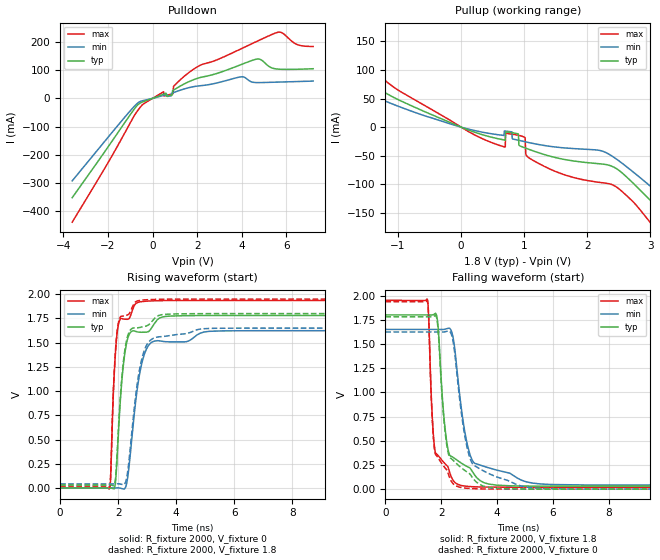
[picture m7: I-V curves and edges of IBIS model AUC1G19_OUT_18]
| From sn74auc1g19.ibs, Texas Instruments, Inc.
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[Model]   AUC1G19_OUT_18
Model_type  Output
Vref =   0
Rref =   2000
Cref =   15p
Vmeas =   0.9
| variable   typ   min   max
C_comp   7.15pF   0.07pF   21.56pF
| C_pullup   7.15pF   0.07pF   21.56pF
| C_pulldown   7.15pF   0.07pF   21.56pF
[Temperature Range]   40   100   -40
| Ambient temperature   25   85   -40
[Voltage range]   1.8   1.65   1.95
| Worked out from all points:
|   slope of the pulldown table from 0 to 0.27 V, typ, clamps not added: 34.4 ohm
|   slope of the pullup table from 0 to 0.27 V, typ, clamps not added: 24.7 ohm
|   rising waveform, R_fixture 2000, V_fixture 0: 20-80 % time 277ps typ, 414ps min, 177ps max; typ from 0 V to 1.78 V
|   falling waveform, R_fixture 2000, V_fixture 1.8: 20-80 % time 326ps typ, 493ps min, 196ps max; typ from 1.8 V to 0.031 V
|   rising waveform, R_fixture 2000, V_fixture 1.8: 20-80 % time 274ps typ, 411ps min, 175ps max; typ from 0.031 V to 1.8 V
|   falling waveform, R_fixture 2000, V_fixture 0: 20-80 % time 330ps typ, 501ps min, 196ps max; typ from 1.78 V to 0 V
[Pulldown]
| AUC1G19_OUT_18
|   Voltage   I(typ)   I(min)   I(max)
-3.6V     -351.5mA   -291.9mA   -438.2mA
-835mV    -39.63mA   -29.64mA   -63.35mA
-410mV    -11.47mA   -7.54mA    -19.84mA
495mV     14.95mA    10.62mA    23.51mA
885mV     12.27mA    19.08mA    15.87mA
925mV     28.56mA    20.18mA    16.89mA
960mV     30.12mA    21.17mA    44.33mA
2.04V     71.79mA    43.96mA    113.2mA
3.925V    118.3mA    76.02mA    173.9mA
4.625V    138.4mA    56.06mA    200mA
5.545V    104.4mA    57.52mA    232.4mA
7.2V      105mA      61.31mA    183.9mA
[Pullup]
| AUC1G19_OUT_18
|   Voltage   I(typ)   I(min)   I(max)
-3.6V     266.7mA    220.9mA    317.6mA
-2.61V    173.9mA    138mA      219.2mA
-2.135V   131.6mA    102.1mA    171.8mA
110mV     -4.812mA   -3.244mA   -7.318mA
695mV     -22.64mA   -6.826mA   -34.84mA
705mV     -8.168mA   -6.941mA   -10.57mA
980mV     -34.9mA    -24.66mA   -16.5mA
1.11V     -40.21mA   -27.81mA   -56.13mA
2.25V     -64.62mA   -42.35mA   -97.29mA
3.1V      -139.4mA   -112.5mA   -180.9mA
3.92V     -232.8mA   -190.6mA   -293.5mA
7.2V      -604.2mA   -510.1mA   -732.1mA
[Ramp]
| AUC1G19_OUT_18
| variable   typ   min   max
dV/dt_r   1.07/2.77E-10   0.98/4.18E-10   1.17/1.77E-10
dV/dt_f   1.07/3.26E-10   0.97/4.96E-10   1.17/1.96E-10
R_load = 2000
[Rising Waveform]
| AUC1G19_OUT_18
R_fixture =   2000
C_fixture =   0
L_fixture =   0
V_fixture =   0
V_fixture_min = 0
V_fixture_max = 0
|   Time   V(typ)   V(min)   V(max)
0s        7.776nV    26.72nV    1.127nV
1.71ns    741.3uV    -20.97uV   -2.097mV
1.89ns    21.41mV    464.4uV    1.311V
1.99ns    458.6mV    1.303mV    1.655V
2.125ns   1.098V     -5.6mV     1.749V
2.275ns   1.472V     23.75mV    1.742V
2.71ns    1.609V     1.124V     1.918V
3.15ns    1.651V     1.502V     1.931V
5.14ns    1.78V      1.617V     1.936V
23ns      1.78V      1.624V     1.936V
[Falling Waveform]
| AUC1G19_OUT_18
R_fixture =   2000
C_fixture =   0
L_fixture =   0
V_fixture =   1.8
V_fixture_min = 1.65
V_fixture_max = 1.95
|   Time   V(typ)   V(min)   V(max)
0s        1.8V       1.65V      1.95V
1.505ns   1.8V       1.65V      1.959V
1.675ns   1.799V     1.65V      777.3mV
1.78ns    1.813V     1.65V      392.8mV
2.225ns   441.9mV    1.66V      237.9mV
2.435ns   327.3mV    1.554V     88.16mV
2.685ns   276.2mV    920.8mV    40.94mV
3.165ns   161mV      275.9mV    24.96mV
5.275ns   31.91mV    62.62mV    19.63mV
23ns      30.96mV    42.25mV    19.48mV
[Rising Waveform]
| AUC1G19_OUT_18
R_fixture =   2000
C_fixture =   0
L_fixture =   0
V_fixture =   1.8
V_fixture_min = 1.65
V_fixture_max = 1.95
|   Time   V(typ)   V(min)   V(max)
0s        30.94mV    42.25mV    19.47mV
1.71ns    31.67mV    42.23mV    18.67mV
1.885ns   48.87mV    42.65mV    1.308V
1.985ns   476.4mV    43.45mV    1.666V
2.115ns   1.097V     37.77mV    1.773V
2.26ns    1.478V     62.82mV    1.781V
2.67ns    1.653V     1.1V       1.931V
3.125ns   1.705V     1.529V     1.945V
4.93ns    1.8V       1.644V     1.95V
23ns      1.8V       1.65V      1.95V
[Falling Waveform]
| AUC1G19_OUT_18
R_fixture =   2000
C_fixture =   0
L_fixture =   0
V_fixture =   0
V_fixture_min = 0
V_fixture_max = 0
|   Time   V(typ)   V(min)   V(max)
0s        1.78V      1.624V     1.936V
1.505ns   1.78V      1.624V     1.944V
1.775ns   1.792V     1.624V     382.7mV
1.88ns    1.677V     1.623V     327.5mV
2.21ns    437.7mV    1.631V     193.8mV
2.42ns    300.1mV    1.537V     59.07mV
2.63ns    243mV      1.011V     23.21mV
3.13ns    115.8mV    259mV      5.595mV
5.03ns    1.275mV    22.59mV    190.4uV
23ns      23.36uV    2.555uV    10.17uV
